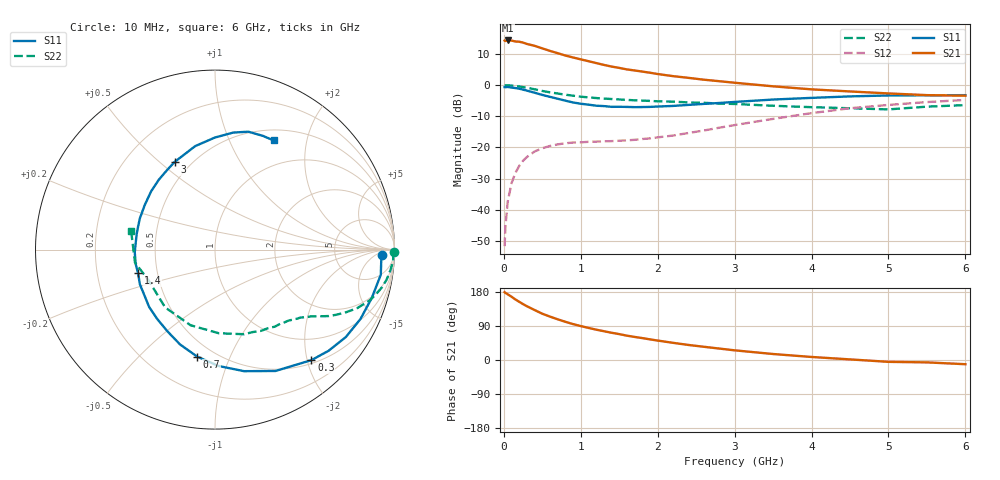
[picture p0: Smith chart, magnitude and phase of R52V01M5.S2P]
! SIEMENS Small Signal Semiconductors
! BFR183
! Si NPN RF Bipolar Junction Transistor in SOT23
! VCE = 2 V  IC = 1.5 mA
! Common Emitter S-Parameters:  May  1996
# GHz  S  MA  R  50
!  f  S11  S21  S12  S22
! GHz  MAG  ANG  MAG  ANG  MAG  ANG  MAG  ANG
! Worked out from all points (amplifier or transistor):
!   36 points, 10 MHz to 6 GHz, reference 50 ohm
!   highest |S21| = 14.3 dB at 50 MHz (marker M1)
!   |S21| within 3 dB of that: start of sweep to 556.2 MHz
!   unconditionally stable (mu >= 1): 1.496 GHz to 2.901 GHz
!   at 250 MHz: K = 0.20, MSG = 19.0 dB, |S12| = -24.3 dB
!   at 1.4 GHz: K = 0.97, MSG = 12.0 dB, |S12| = -18.0 dB
!   at 6 GHz: K = 0.94, MSG = 0.7 dB, |S12| = -4.8 dB
!   S11 on the Smith chart (normalised r, x): 10 MHz: 23, -10; 300 MHz: 0.56, -2.08; 700 MHz: 0.41, -0.76; 1.4 GHz: 0.39, -0.13; 3 GHz: 0.41, +0.56; 6 GHz: 0.64, +1.48
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0.01  0.93 -1.8  5.197 179.0  0.0026 89.2  0.9973 -0.7
0.02  0.928 -3.3  5.1 177.3  0.0052 85.4  0.9931 -1.4
0.05  0.9343 -8.6  5.216 173.4  0.0134 85.1  0.9944 -3.5
0.1  0.9142 -17.1  5.19 167.0  0.0267 80.4  0.9842 -6.7
0.15  0.898 -25.5  5.022 159.8  0.0389 75.4  0.9705 -10.0
0.2  0.877 -33.7  4.978 153.6  0.0505 70.9  0.9525 -12.9
0.25  0.8474 -41.7  4.816 147.5  0.0612 66.1  0.9286 -15.8
0.3  0.8173 -48.9  4.586 141.8  0.0702 62.8  0.9068 -18.2
0.4  0.7556 -63.5  4.276 131.9  0.0861 55.8  0.8576 -22.3
0.5  0.6963 -76.6  3.891 122.1  0.097 50.4  0.8073 -25.7
0.6  0.6485 -88.3  3.545 114.5  0.1056 46.0  0.7662 -28.3
0.7  0.6046 -99.4  3.26 107.4  0.1119 42.6  0.7339 -30.3
0.9  0.5271 -120.1  2.781 94.7  0.1199 38.5  0.6769 -33.3
1.1  0.4865 -139.0  2.424 84.7  0.1231 36.9  0.6361 -36.2
1.4  0.4484 -162.9  1.988 71.9  0.1262 37.4  0.599 -39.9
1.7  0.4433 174.8  1.72 60.9  0.1324 41.3  0.5707 -43.8
2.2  0.4639 147.4  1.395 45.3  0.1552 48.8  0.5439 -52.1
3  0.5378 114.7  1.093 25.5  0.2285 53.7  0.4986 -71.0
3.5  0.5872 100.8  0.957 15.8  0.2874 51.0  0.4665 -87.4
4.5  0.6597 81.2  0.792 1.6  0.426 38.5  0.4253 -130.8
5.5  0.6875 67.2  0.691 -6.3  0.5349 23.1  0.4515 -170.7
6  0.6906 61.7  0.677 -11.1  0.5786 13.5  0.4783 167.7
